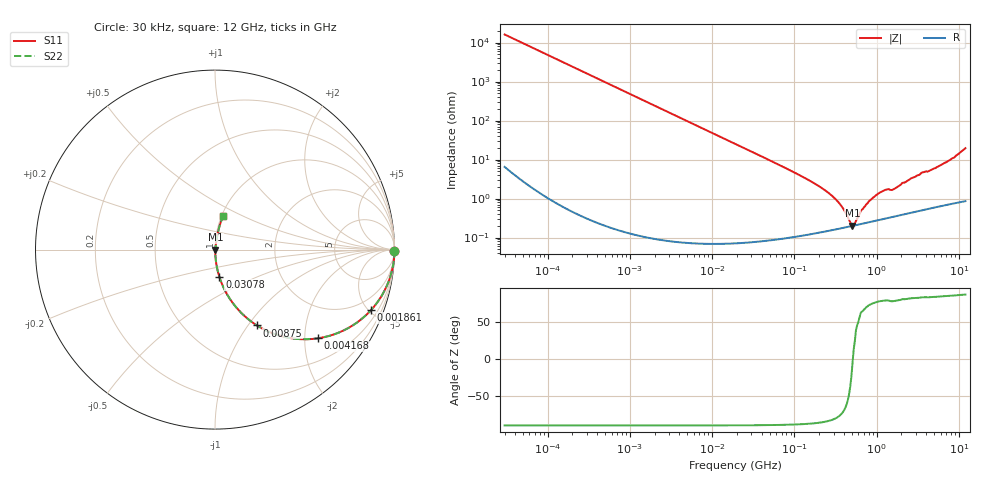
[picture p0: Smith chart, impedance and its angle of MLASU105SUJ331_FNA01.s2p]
! MLASU105SUJ331_FNA01  S-PARAMETER MODEL  ( General Type )
! Model Generated by TAIYO YUDEN Corporation (http://www.ty-top.com)
! Version 4.0
! TAIYO YUDEN Control No. 120810
! Copyright(c) 2003 TAIYO YUDEN CO.,LTD. All Rights Reserved.
! Product Description (link to TY-COMPAS)
! https://ds.yuden.co.jp/TYCOMPAS/or/detail?pn=MLASU105SUJ331JFNA01&u=M
! Products Name : Multilayer Ceramic Capacitors
! Characteristics :
!  Capacitance : 330 pF , Rated Voltage : 50V , TCC : UJ / U2J
!  Case Size : 1.0 x 0.5 / 0.039 x 0.02 [mm/inch] , Thickness : 0.5 / 0.02 [mm/inch]
!  (Conditions: Temperature = 25 degC , DC Bias Current/Voltage = 0A / 0V)
! External Node Assignments :
!  1  o---| |---o  2
! GND o---------o GND
! Frequency Range : 0.03MHz  -  12000MHz  [ 401 STEP ]
# MHz S RI R 50
! Freq[MHz].  S11 Real  S11 Imag  S21 Real  S21 Imag  S12 Real  S12 Imag  S22 Real  S22 Imag
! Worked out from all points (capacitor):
!   401 points, 30 kHz to 12 GHz, reference 50 ohm
!   read as one part in series: C = 330 pF near 32 kHz
!   lowest |Z| = 200 mohm at 509 MHz (marker M1)
!   series resonance near 514.4 MHz, so ESL is about 290 pH
!   S11 on the Smith chart (normalised r, x): 30 kHz: open; 1.861 MHz: 1.00, -5.19; 4.168 MHz: 1.00, -2.32; 8.75 MHz: 1.00, -1.10; 30.78 MHz: 1.00, -0.31; 12 GHz: 1.02, +0.39
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0.03  1 -0.00621  4.11e-05 0.00621  4.11e-05 0.00621  1 -0.00621
0.260295  0.9971 -0.0537  0.00291 0.0537  0.00291 0.0537  0.9971 -0.0537
0.730518  0.9776 -0.1479  0.0224 0.1479  0.0224 0.1479  0.9776 -0.1479
1.861146  0.8706 -0.3355  0.1294 0.3355  0.1294 0.3355  0.8706 -0.3355
2.258455  0.8204 -0.3836  0.1796 0.3836  0.1796 0.3836  0.8204 -0.3836
4.167822  0.5731 -0.4943  0.4269 0.4943  0.4269 0.4943  0.5731 -0.4943
8.750395  0.2337 -0.4225  0.7663 0.4225  0.7663 0.4225  0.2337 -0.4225
18.97367  0.0613 -0.2384  0.9387 0.2384  0.9387 0.2384  0.0613 -0.2384
30.77716  0.0246 -0.1524  0.9754 0.1524  0.9754 0.1524  0.0246 -0.1524
164.6252  0.00192 -0.0263  0.9981 0.0263  0.9981 0.0263  0.00192 -0.0263
324.0443  0.0017 -0.00901  0.9983 0.00901  0.9983 0.00901  0.0017 -0.00901
380.7415  0.00177 -0.00578  0.9982 0.00578  0.9982 0.00578  0.00177 -0.00578
508.9517  0.00198 -0.000217  0.998 0.000217  0.998 0.000217  0.00198 -0.000217
560.6502  0.00207 0.00167  0.9979 -0.00167  0.9979 -0.00167  0.00207 0.00167
680.3351  0.00229 0.00487  0.9977 -0.00487  0.9977 -0.00487  0.00229 0.00487
852.6267  0.0026 0.00898  0.9974 -0.00898  0.9974 -0.00898  0.0026 0.00898
1139.739  0.0031 0.0144  0.9969 -0.0144  0.9969 -0.0144  0.0031 0.0144
1428.372  0.0035 0.0167  0.9965 -0.0167  0.9965 -0.0167  0.0035 0.0167
1625.032  0.00371 0.017  0.9963 -0.017  0.9963 -0.017  0.00371 0.017
3639.072  0.00717 0.0462  0.9928 -0.0462  0.9928 -0.0462  0.00717 0.0462
5534.236  0.0102 0.064  0.9898 -0.064  0.9898 -0.064  0.0102 0.064
12000  0.0444 0.1852  0.9556 -0.1852  0.9556 -0.1852  0.0444 0.1852
